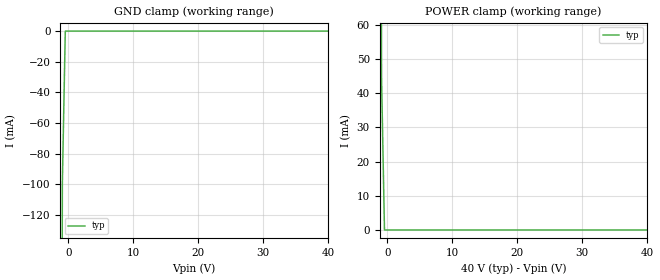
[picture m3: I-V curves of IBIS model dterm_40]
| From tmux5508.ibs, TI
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| dterm_40
[Model]   dterm_40
Model_type   Terminator
|   typ   min   max
C_comp   6.362683e-12   NA   NA
[Voltage Range]   40   NA   NA
[Temperature Range]   27   NA   NA
[Power Clamp Reference]   40   NA   NA
[GND Clamp Reference]   0   NA   NA
[GND Clamp]
|   Voltage   I(typ)   I(min)   I(max)
-5V       -13.02A    NA         NA
-1.364V   -1.178A    NA         NA
-909.1mV  -99.73mA   NA         NA
-454.5mV  -820.3nA   NA         NA
40V       660nA      NA         NA
[POWER Clamp]
|   Voltage   I(typ)   I(min)   I(max)
-5V       8.45A      NA         NA
-1.364V   585.4mA    NA         NA
-909.1mV  44.73mA    NA         NA
-454.5mV  673.7nA    NA         NA
40V       -4.292nA   NA         NA
